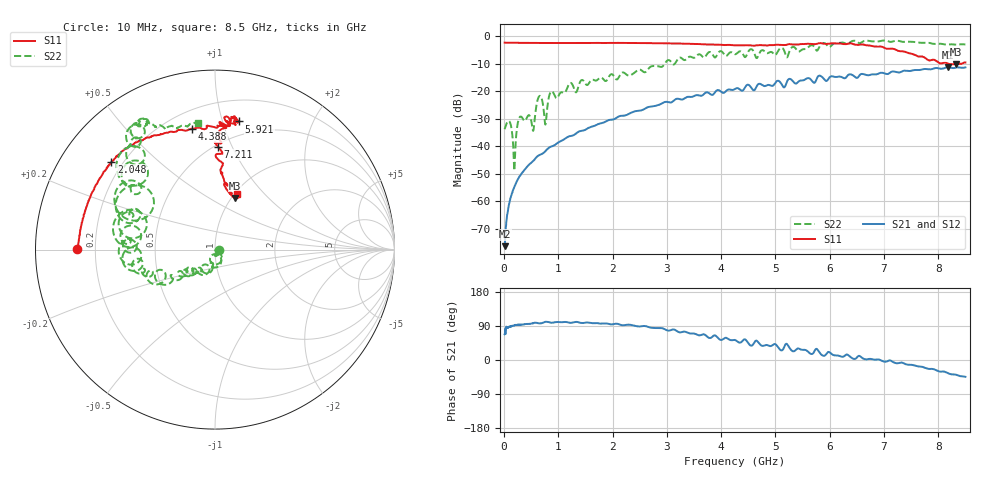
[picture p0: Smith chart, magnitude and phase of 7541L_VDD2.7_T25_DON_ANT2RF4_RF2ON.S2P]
!Agilent Technologies,E5071C,MY46417908,A.11.23
!Date: Wed Dec 09 17:17:47 2020
!Data & Calibration Information:
!Freq	S11:SOLT2(ON)	S21:SOLT2(ON)	S12:SOLT2(ON)	S22:SOLT2(ON)
!PortZ  Port1:50+j0  Port2:50+j0
!Above PortZ is port z conversion or system Z0 setting when saving the data.
!When reading, reference impedance value at option line is always used.
# Hz S dB R 50
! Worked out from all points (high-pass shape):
!   1601 points, 10 MHz to 8.5 GHz, reference 50 ohm
!   highest |S21| = -11.28 dB at 8.182 GHz (marker M1); lowest = -76.3 dB at 10 MHz (marker M2)
!   |S21| within 3 dB of the highest: 6.33 GHz to 6.434 GHz (104.1 MHz wide, 1.63 % of centre); 6.546 GHz to end of sweep
!   lowest |S11| = -10.2 dB at 8.33 GHz (marker M3), VSWR 1.89, Z = 51.8 + j32.9 ohm
!   |S11| at or under -10 dB: 8.188 GHz to 8.38 GHz (192 MHz wide, 2.32 % of centre); 8.408986 GHz to 8.426541 GHz (17.55 MHz wide, 0.209 % of centre)
!   |S22| runs from -48.8 to -1.5 dB; largest |S21 - S12| = 0.0024
!   S11 on the Smith chart (normalised r, x): 10 MHz: 0.13, +0.00; 2.048 GHz: 0.16, +0.36; 4.388 GHz: 0.31, +0.78; 5.921 GHz: 0.37, +1.13; 7.211 GHz: 0.52, +0.88; 8.5 GHz: 1.03, +0.72
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1e7  -2.30 179.7  -76.27 68.0  -79.49 68.6  -33.77 -0.2
1.002062e8  -2.36 177.9  -60.43 88.2  -60.23 88.3  -30.96 -53.1
1.904125e8  -2.38 175.9  -54.71 90.8  -54.64 91.4  -48.84 -40.6
2.965375e8  -2.40 173.8  -50.64 93.1  -50.65 92.8  -29.19 -48.4
5.300125e8  -2.42 169.0  -45.39 97.1  -45.40 97.0  -34.10 -78.3
6.520562e8  -2.43 166.8  -43.17 96.6  -43.13 96.8  -21.71 -80.8
7.634875e8  -2.45 164.4  -41.70 100.8  -41.69 100.6  -32.08 -84.9
8.696125e8  -2.44 162.1  -40.03 98.3  -40.06 98.3  -20.03 -87.4
1.426769e9  -2.44 151.4  -34.36 97.5  -34.36 97.5  -15.93 -118.4
2.0476e9  -2.43 139.8  -29.95 95.6  -29.94 95.6  -15.23 -145.7
2.843538e9  -2.51 129.2  -25.00 84.3  -25.00 84.3  -10.92 -150.1
4.255e9  -3.32 103.7  -19.12 52.8  -19.12 52.8  -6.52 174.1
4.387656e9  -3.28 100.7  -19.79 49.5  -19.80 49.4  -6.05 164.5
5.14645e9  -3.20 84.0  -18.45 29.6  -18.43 29.6  -4.67 142.2
5.247269e9  -2.86 84.6  -15.53 34.7  -15.52 34.8  -6.06 160.8
5.671769e9  -2.81 80.1  -16.17 15.8  -16.12 15.7  -3.26 136.2
5.921162e9  -2.77 79.4  -16.09 13.0  -16.04 13.1  -2.66 128.6
7.088538e9  -4.54 88.2  -13.56 -1.4  -13.61 -1.5  -1.90 118.3
7.210581e9  -4.83 88.3  -12.91 -8.0  -12.92 -7.7  -1.64 120.5
8.181625e9  -9.94 73.8  -11.28 -34.9  -11.31 -34.9  -2.96 106.9
8.3302e9  -10.23 68.9  -11.37 -39.0  -11.37 -39.0  -3.07 102.6
8.5e9  -9.53 68.1  -11.31 -44.3  -11.38 -44.2  -2.98 97.7
